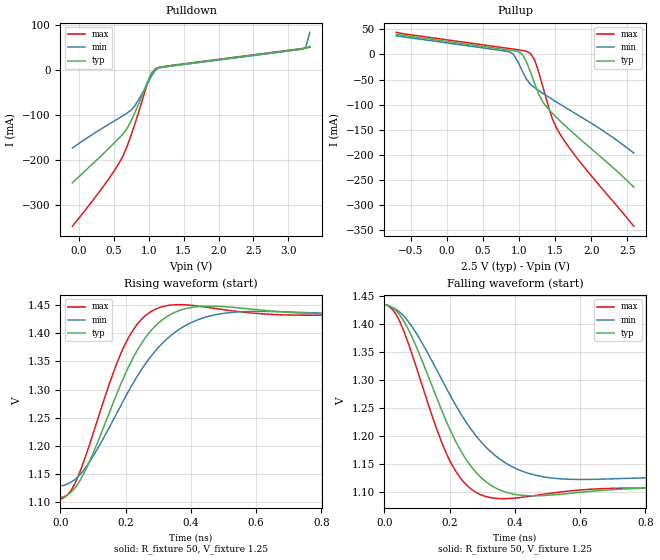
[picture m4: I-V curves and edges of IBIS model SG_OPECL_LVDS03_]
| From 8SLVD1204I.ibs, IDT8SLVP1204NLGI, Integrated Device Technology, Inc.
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| 3.16407e+00   -1.31771e-02   -1.64528e+00   -2.08013e-04
| 3.23015e+00   -1.68690e-01   -1.66048e+01   -1.45006e-03
| 3.29623e+00   -2.17012e+00   -1.80319e+02   -1.73913e-02
| 3.36231e+00   -2.12126e+01   -2.25699e+03   -2.22512e-01
| 3.42839e+00   -2.36334e+02   -2.89472e+04   -2.86202e+00
| 3.49447e+00   -2.97463e+03   -3.72391e+05   -2.72019e+01
| 3.56055e+00   -3.81771e+04   -1.39023e+06   -3.10131e+02
| 3.62663e+00   -4.81523e+05   -2.47550e+06   -3.92107e+03
| 3.69271e+00   -1.50194e+06   -4.41843e+06   -5.03512e+04
| 3.75879e+00   -2.61026e+06   -1.16364e+07   -5.91499e+05
| 3.82487e+00   -4.84984e+06   -2.00037e+07   -1.61428e+06
| 3.89095e+00   -1.25431e+07   -2.83711e+07   -2.75300e+06
| 3.95703e+00   -2.09105e+07   -3.67385e+07   -5.38384e+06
| 4.02311e+00   -2.92779e+07   -4.51059e+07   -1.34498e+07
| 4.08920e+00   -3.76452e+07   -5.34733e+07   -2.18172e+07
| 4.15528e+00   -4.60126e+07   -6.18406e+07   -3.01846e+07
| 4.22136e+00   -5.43800e+07   -7.02080e+07   -3.85520e+07
| 4.28744e+00   -6.27474e+07   -7.85754e+07   -4.69194e+07
| 4.35352e+00   -7.11148e+07   -8.69428e+07   -5.52868e+07
| 4.41960e+00   -7.94822e+07   -9.53102e+07   -6.36541e+07
| 4.48568e+00   -8.78495e+07   -1.03678e+08   -7.20215e+07
| 4.55176e+00   -9.62169e+07   -1.12045e+08   -8.03889e+07
| 4.61784e+00   -1.04584e+08   -1.20412e+08   -8.87563e+07
| 4.68392e+00   -1.12952e+08   -1.28780e+08   -9.71237e+07
| 4.75000e+00   -1.21319e+08   -1.37147e+08   -1.05491e+08
| 4.75100e+00   -1.21446e+08   -1.37274e+08   -1.05618e+08
| 4.80080e+00   -1.27752e+08   -1.43580e+08   -1.11924e+08
| 4.85060e+00   -1.34057e+08   -1.49885e+08   -1.18229e+08
| 4.90040e+00   -1.40363e+08   -1.56191e+08   -1.24535e+08
| 4.95020e+00   -1.46669e+08   -1.62497e+08   -1.30841e+08
| 5.00000e+00   -1.52975e+08   -1.68803e+08   -1.37147e+08
[Model]   SG_OPECL_LVDS03_
Model_type   Output
Polarity   Non-Inverting
|   typ   min   max
C_comp   2pF   1.5pF   2.5pF
Vmeas = 1.271V
Rref = 50
Cref = 0
Vref = 1.271V
|   typ   min   max
[Voltage range]   2.5V   2.375V   2.625V
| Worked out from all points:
|   slope of the pulldown table from 0 to 0.375 V, typ, clamps not added: 6.82 ohm
|   slope of the pullup table from 0 to 0.375 V, typ, clamps not added: 49.9 ohm
|   rising waveform, R_fixture 50, V_fixture 1.25: 20-80 % time 145ps typ, 188ps min, 118ps max; typ from 1.11 V to 1.44 V
|   falling waveform, R_fixture 50, V_fixture 1.25: 20-80 % time 145ps typ, 188ps min, 118ps max; typ from 1.43 V to 1.11 V
[Pulldown]
|Voltage   I (typ)   I (min)   I (max)
|Note, modeling breaks down at 250mA and above.  This is well beyond the functional   |
|operating range of the device.  Should this scenario occur, catastrophic failure and   |
|possible damage to the device and/or board is of higher concern than the I-V curve   |
|behavior.  The IBIS checker will flag currents in excess of 10A with warnings.  Lines   |
|with currents in excess of 0.35 A have been commented out.  The points still remain|
|available to the user if the user desires to use them.   |
|-2.14000e+00   -1.08219e+08   -1.43135e+08   -8.74828e+07
|-1.78000e+00   -6.23289e+07   -8.44505e+07   -4.92803e+07
|-1.42000e+00   -1.64384e+07   -2.57662e+07   -1.10777e+07
|-1.06000e+00   -3.61589e+04   -1.00624e+04   -8.67977e+04
|-7.00000e-01   -3.88144e-01   -2.41880e-01   -1.66220e+00
|-6.90000e-01   -3.71316e-01   -2.40639e-01   -1.33634e+00
|-6.30345e-01   -3.32587e-01   -2.33737e-01   -5.94847e-01
|-5.70690e-01   -3.20589e-01   -2.27008e-01   -4.70441e-01
|-5.11034e-01   -3.11631e-01   -2.20303e-01   -4.37048e-01
|-4.51379e-01   -3.03054e-01   -2.13615e-01   -4.19102e-01
|-3.91724e-01   -2.94523e-01   -2.06948e-01   -4.05511e-01
|-3.32069e-01   -2.85983e-01   -2.00304e-01   -3.93643e-01
|-2.72414e-01   -2.77420e-01   -1.93688e-01   -3.82290e-01
|-2.12759e-01   -2.68830e-01   -1.87106e-01   -3.71015e-01
|-1.53103e-01   -2.60215e-01   -1.80562e-01   -3.59699e-01
-93.45mV  -251.6mA   -174.1mA   -348.3mA
383.8mV   -181.7mA   -125.6mA   -252.4mA
622.4mV   -144.3mA   -103.1mA   -194.9mA
682.1mV   -132.8mA   -97.16mA   -174.2mA
801.4mV   -95.86mA   -80.35mA   -121mA
980.3mV   -27.81mA   -31.57mA   -31.15mA
1.04V     -7.483mA   -13.85mA   -7.817mA
1.1V      2.656mA    -101.8uA   2.755mA
1.219V    6.878mA    5.991mA    7.537mA
3.188V    46.4mA     45.58mA    47.08mA
3.247V    47.87mA    48.51mA    48.35mA
3.307V    51.85mA    83.43mA    50.03mA
| 3.36655e+00   8.13204e-02   7.41351e-01   5.45059e-02
| 3.42621e+00   3.70775e-01   1.27593e+01   7.83695e-02
| 3.48586e+00   3.31085e+00   2.13018e+02   2.36163e-01
| 3.54552e+00   2.92934e+01   4.05877e+03   1.31939e+00
| 3.60517e+00   2.73514e+02   7.89116e+04   8.57624e+00
| 3.66483e+00   2.74211e+03   1.53684e+06   5.14192e+01
| 3.72448e+00   2.78895e+04   9.61928e+06   3.36030e+02
| 3.78414e+00   2.84259e+05   1.81665e+07   2.29124e+03
| 3.84379e+00   2.89799e+06   2.67137e+07   1.57902e+04
| 3.90345e+00   9.58180e+06   3.52609e+07   1.09055e+05
| 3.96310e+00   1.62656e+07   4.38080e+07   7.53499e+05
| 4.02276e+00   2.29494e+07   5.23552e+07   4.58446e+06
| 4.08241e+00   2.96332e+07   6.09024e+07   1.01485e+07
| 4.14207e+00   3.63170e+07   6.94496e+07   1.57126e+07
| 4.20172e+00   4.30008e+07   7.79968e+07   2.12767e+07
| 4.26138e+00   4.96846e+07   8.65440e+07   2.68408e+07
| 4.32103e+00   5.63684e+07   9.50912e+07   3.24049e+07
| 4.38069e+00   6.30523e+07   1.03638e+08   3.79690e+07
| 4.44034e+00   6.97361e+07   1.12186e+08   4.35331e+07
| 4.50000e+00   7.64199e+07   1.20733e+08   4.90971e+07
| 4.51000e+00   7.75403e+07   1.22166e+08   5.00298e+07
| 4.60800e+00   8.85203e+07   1.36207e+08   5.91704e+07
| 4.70600e+00   9.95002e+07   1.50248e+08   6.83109e+07
| 4.80400e+00   1.10480e+08   1.64289e+08   7.74515e+07
| 4.90200e+00   1.21460e+08   1.78330e+08   8.65920e+07
| 5.00000e+00   1.32440e+08   1.92371e+08   9.57325e+07
[Pullup]
|Voltage   I (typ)   I (min)   I (max)
|Note, modeling breaks down at 250mA and above.  This is well beyond the functional   |
|operating range of the device.  Should this scenario occur, catastrophic failure and   |
|possible damage to the device and/or board is of higher concern than the I-V curve   |
|behavior.  The IBIS checker will flag currents in excess of 10A with warnings.  Lines   |
|with currents in excess of 0.35 A have been commented out.  The points still remain|
|available to the user if the user desires to use them.   |
|-2.14000e+00   9.21056e+07   1.22882e+08   7.38139e+07
|-1.78000e+00   5.17709e+07   7.13023e+07   4.02364e+07
|-1.42000e+00   1.14363e+07   1.97228e+07   6.65893e+06
|-1.06000e+00   4.97692e+01   1.90536e+01   9.61909e+01
-700mV    40.11mA    37.09mA    44.23mA
861mV     8.756mA    5.492mA    11.93mA
920.7mV   7.515mA    684.1uA    10.73mA
1.04V     1.214mA    -31mA      8.245mA
1.1V      -13.26mA   -48.34mA   6.5mA
1.159V    -35.53mA   -59.88mA   2.075mA
1.219V    -58.99mA   -66.53mA   -11.82mA
1.338V    -96.55mA   -78.16mA   -68.5mA
1.458V    -116.6mA   -89.14mA   -126.6mA
1.577V    -133.6mA   -99.85mA   -160.9mA
1.875V    -172.3mA   -126.1mA   -219.7mA
2.591V    -264.5mA   -196.5mA   -342.7mA
| 2.65069e+00   -2.72894e-01   -2.03008e-01   -3.53526e-01
| 2.71034e+00   -2.81279e-01   -2.09598e-01   -3.64391e-01
| 2.77000e+00   -2.89674e-01   -2.16215e-01   -3.75266e-01
| 2.82966e+00   -2.98071e-01   -2.22854e-01   -3.86128e-01
| 2.88931e+00   -3.06464e-01   -2.29512e-01   -3.96966e-01
| 2.94897e+00   -3.14850e-01   -2.36187e-01   -4.07775e-01
| 3.00862e+00   -3.23248e-01   -2.42884e-01   -4.18576e-01
| 3.06828e+00   -3.31855e-01   -2.49761e-01   -4.29543e-01
| 3.12793e+00   -3.42729e-01   -2.59900e-01   -4.41902e-01
| 3.18759e+00   -3.76842e-01   -3.33345e-01   -4.64139e-01
| 3.24724e+00   -6.48029e-01   -1.63967e+00   -5.54887e-01
| 3.30690e+00   -3.33436e+00   -2.06497e+01   -1.11929e+00
| 3.36655e+00   -2.31891e+01   -3.39768e+02   -4.82520e+00
| 3.42621e+00   -2.04076e+02   -6.49922e+03   -2.37250e+01
| 3.48586e+00   -2.02664e+03   -1.26384e+05   -1.42739e+02
| 3.54552e+00   -2.05831e+04   -1.12384e+06   -9.53500e+02
| 3.60517e+00   -2.09733e+05   -2.37601e+06   -6.54397e+03
| 3.66483e+00   -1.06686e+06   -5.01126e+06   -4.51548e+04
| 3.72448e+00   -2.01265e+06   -1.42710e+07   -3.11930e+05
| 3.78414e+00   -3.18967e+06   -2.39955e+07   -1.06966e+06
| 3.84379e+00   -6.72405e+06   -3.37200e+07   -1.84957e+06
| 3.90345e+00   -1.43285e+07   -4.34445e+07   -2.70925e+06
| 3.96310e+00   -2.19330e+07   -5.31690e+07   -4.12011e+06
| 4.02276e+00   -2.95374e+07   -6.28936e+07   -8.71749e+06
| 4.08241e+00   -3.71419e+07   -7.26181e+07   -1.50480e+07
| 4.14207e+00   -4.47463e+07   -8.23426e+07   -2.13785e+07
| 4.20172e+00   -5.23508e+07   -9.20671e+07   -2.77090e+07
| 4.26138e+00   -5.99552e+07   -1.01792e+08   -3.40395e+07
| 4.32103e+00   -6.75597e+07   -1.11516e+08   -4.03700e+07
| 4.38069e+00   -7.51642e+07   -1.21241e+08   -4.67005e+07
| 4.44034e+00   -8.27686e+07   -1.30965e+08   -5.30310e+07
| 4.50000e+00   -9.03731e+07   -1.40690e+08   -5.93615e+07
| 4.51000e+00   -9.16478e+07   -1.42320e+08   -6.04227e+07
| 4.60800e+00   -1.04140e+08   -1.58295e+08   -7.08223e+07
| 4.70600e+00   -1.16633e+08   -1.74270e+08   -8.12218e+07
| 4.80400e+00   -1.29125e+08   -1.90245e+08   -9.16214e+07
| 4.90200e+00   -1.41617e+08   -2.06220e+08   -1.02021e+08
| 5.00000e+00   -1.54110e+08   -2.22196e+08   -1.12421e+08
[Ramp]
|   typ   min   max
dV/dt_r   0.204/0.154n   0.186/0.193n   0.207/0.126n
dV/dt_f   0.204/0.154n   0.186/0.193n   0.207/0.126n
R_load =   50.0000
[Rising Waveform]
R_fixture = 50
V_fixture = 1.25   |Vcc_typ
V_fixture_min = 1.25 |Vcc_min
V_fixture_max = 1.25 |Vcc_max
C_fixture = 0.0p
| Time   typ   min   max
0s        1.108V     1.129V     1.106V
35.03ps   1.119V     1.136V     1.123V
70.07ps   1.149V     1.156V     1.17V
160.2ps   1.274V     1.244V     1.327V
207.7ps   1.339V     1.296V     1.391V
257.8ps   1.39V      1.344V     1.43V
320.3ps   1.427V     1.387V     1.449V
425.4ps   1.448V     1.425V     1.448V
565.6ps   1.444V     1.439V     1.437V
2.498ns   1.435V     1.434V     1.435V
[Falling Waveform]
R_fixture = 50
V_fixture = 1.25   |Vcc_typ
V_fixture_min = 1.25 |Vcc_min
V_fixture_max = 1.25 |Vcc_max
C_fixture = 0.0p
| Time   typ   min   max
0s        1.434V     1.433V     1.434V
35.03ps   1.424V     1.426V     1.417V
70.07ps   1.394V     1.406V     1.37V
160.2ps   1.268V     1.318V     1.213V
207.7ps   1.203V     1.266V     1.149V
257.8ps   1.152V     1.219V     1.11V
320.3ps   1.115V     1.175V     1.091V
425.4ps   1.095V     1.137V     1.092V
565.6ps   1.098V     1.123V     1.103V
2.498ns   1.107V     1.128V     1.105V
